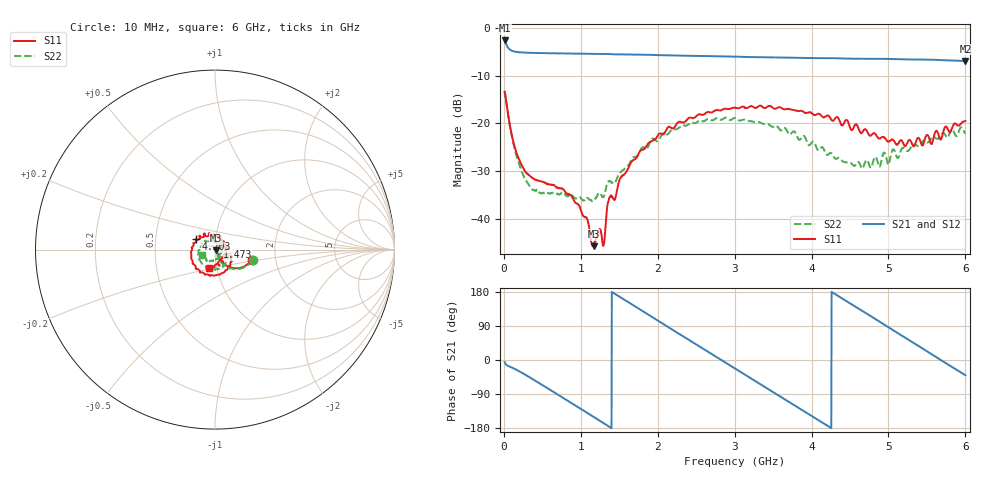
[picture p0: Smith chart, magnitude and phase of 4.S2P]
!Agilent Technologies,E5071C,MY46316741,A.11.02
!Date: Thu Jul 30 16:12:17 2020
!Data & Calibration Information:
!Freq	S11:SOLT4(ON)	S21:SOLT4(ON)	S12:SOLT4(ON)	S22:SOLT4(ON)
!PortZ  Port1:50+j0  Port2:50+j0
!Above PortZ is port z conversion or system Z0 setting when saving the data.
!When reading, reference impedance value at option line is always used.
# Hz S dB R 50
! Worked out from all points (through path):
!   1561 points, 10 MHz to 6 GHz, reference 50 ohm
!   highest |S21| = -2.66 dB at 10 MHz (marker M1); lowest = -7.0 dB at 6 GHz (marker M2)
!   group delay of S21, straight-line fit = 350 ps
!   lowest |S11| = -45.7 dB at 1.166 GHz (marker M3), VSWR 1.01, Z = 50.4 - j0.313 ohm
!   |S11| at or under -10 dB: start of sweep to end of sweep
!   |S22| runs from -36.3 to -13.2 dB; largest |S21 - S12| = 0.0073
!   S11 on the Smith chart (normalised r, x): 10 MHz: 1.51, -0.18; 1.473 GHz: 1.03, +0.03; 4.203 GHz: 0.80, +0.09; 6 GHz: 0.92, -0.19
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1e7  -13.39 -15.1  -2.66 -5.4  -2.65 -5.4  -13.24 -15.5
1.559103e8  -25.80 -62.2  -5.04 -24.9  -5.03 -24.9  -26.30 -68.2
3.440577e8  -31.10 -50.7  -5.25 -46.7  -5.24 -46.8  -33.36 -51.4
6.819551e8  -33.37 -47.4  -5.35 -88.8  -5.35 -88.9  -34.59 -27.2
1.012173e9  -38.65 -55.4  -5.43 -130.5  -5.43 -130.7  -35.91 -14.6
1.165763e9  -45.73 -36.9  -5.47 -150.0  -5.47 -150.2  -36.22 -3.6
1.238718e9  -42.33 29.3  -5.48 -159.2  -5.47 -159.4  -34.60 10.5
1.296314e9  -45.53 38.2  -5.48 -166.5  -5.47 -166.7  -35.35 6.3
1.365429e9  -35.90 39.0  -5.50 -175.5  -5.50 -175.8  -32.18 12.2
1.472942e9  -33.90 39.8  -5.58 170.9  -5.57 170.6  -31.47 13.8
1.66109e9  -28.03 35.5  -5.63 147.3  -5.62 147.0  -27.60 12.3
2.006667e9  -22.44 3.8  -5.73 103.3  -5.72 103.1  -23.65 -15.3
2.271609e9  -19.74 -22.6  -5.82 69.9  -5.81 69.4  -21.01 -40.1
2.571109e9  -18.22 -49.8  -5.91 32.2  -5.91 31.8  -19.49 -68.9
3.005e9  -16.75 -91.0  -6.04 -22.6  -6.04 -23.1  -18.87 -116.0
3.508006e9  -16.89 -139.2  -6.22 -85.8  -6.20 -86.3  -20.73 -173.5
4.007173e9  -17.94 173.5  -6.35 -148.4  -6.33 -149.0  -23.94 121.1
4.203e9  -18.37 151.2  -6.36 -173.0  -6.35 -173.6  -26.65 94.3
4.563936e9  -20.40 109.0  -6.50 141.6  -6.50 140.8  -28.86 24.4
5.001667e9  -23.84 49.0  -6.52 86.2  -6.52 85.4  -28.69 -43.3
5.527712e9  -23.06 -37.3  -6.68 19.4  -6.67 18.7  -23.86 -107.6
6e9  -19.53 -107.3  -6.96 -40.1  -6.94 -41.0  -22.15 -159.1
